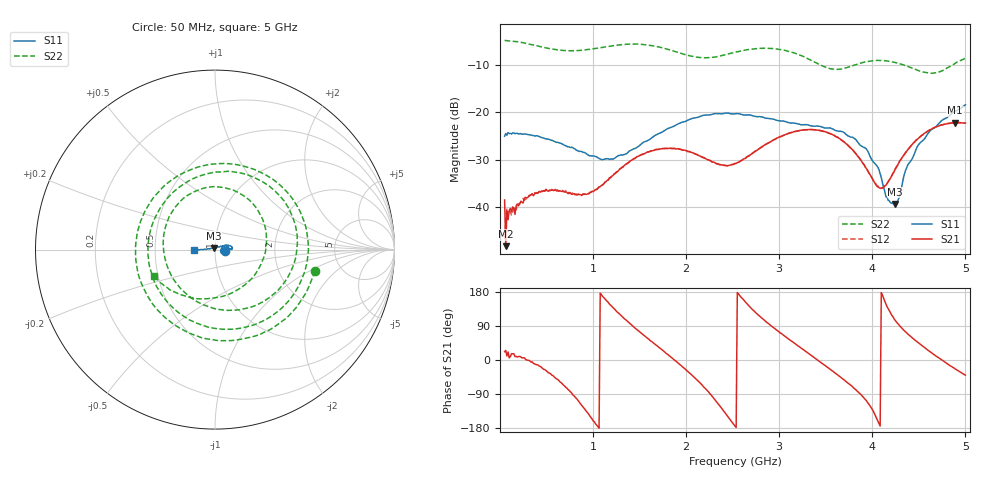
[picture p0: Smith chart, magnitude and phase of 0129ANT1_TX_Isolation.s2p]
! MASWSS0129 de-embedded Sparameters using port extention method. ANT1 to TX Isolation using 3 volt control
! 100pF blocking capacitor
! Sample board 1000013136
# Hz  S  DB  R  50
! Freq  S11  S21  S12  S22
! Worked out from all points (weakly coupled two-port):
!   401 points, 50 MHz to 5 GHz, reference 50 ohm
!   highest |S21| = -22.22 dB at 4.889 GHz (marker M1); lowest = -48.2 dB at 62.38 MHz (marker M2)
!   lowest |S11| = -39.3 dB at 4.245 GHz (marker M3), VSWR 1.02, Z = 49.3 + j0.817 ohm
!   |S11| at or under -10 dB: start of sweep to end of sweep
!   |S22| runs from -11.8 to -4.9 dB; largest |S21 - S12| = 0.009
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5e7  -25.07 -6.4  -38.48 21.8  -46.68 -19.8  -4.91 -12.0
6.2375e7  -24.50 -3.5  -48.21 25.2  -42.16 8.2  -4.94 -14.8
2.48e8  -24.63 -12.8  -39.14 5.6  -38.17 5.5  -5.41 -58.7
4.08875e8  -25.06 -18.4  -37.04 -13.3  -36.95 -14.3  -6.06 -98.4
6.44e8  -26.52 -26.4  -36.55 -57.7  -36.51 -57.0  -6.94 -159.2
8.79125e8  -28.31 -27.3  -37.42 -119.8  -37.55 -119.2  -6.96 140.1
1.12663e9  -29.90 -12.4  -34.75 161.5  -34.86 162.2  -6.29 80.7
1.3865e9  -28.25 12.1  -30.50 98.5  -30.52 98.1  -5.69 22.1
1.70825e9  -24.50 23.0  -27.80 33.4  -27.77 32.8  -6.30 -51.3
1.90625e9  -22.57 19.0  -27.69 -6.5  -27.70 -6.8  -7.41 -100.4
2.14138e9  -20.98 12.2  -29.17 -58.5  -29.12 -59.0  -8.48 -165.2
2.525e9  -20.34 2.7  -30.81 -174.0  -30.83 -173.7  -7.40 94.4
2.723e9  -20.81 1.3  -28.53 130.8  -28.47 130.7  -6.71 54.3
2.95813e9  -21.63 3.0  -25.67 81.7  -25.67 81.5  -6.66 9.4
3.35413e9  -22.95 13.9  -23.66 10.3  -23.69 10.3  -9.20 -77.6
3.72538e9  -24.80 23.5  -26.74 -58.3  -26.72 -58.3  -10.63 167.6
4.0595e9  -31.59 34.0  -35.74 -160.4  -35.57 -160.3  -9.09 91.2
4.18325e9  -38.68 65.2  -34.28 129.6  -34.28 129.6  -9.33 65.9
4.24513e9  -39.30 130.2  -32.04 105.0  -31.98 104.9  -9.55 52.6
4.49263e9  -26.98 175.5  -25.56 45.8  -25.53 45.6  -11.23 -10.0
4.88863e9  -19.86 -178.9  -22.22 -23.3  -22.23 -23.4  -9.76 -132.9
5e9  -18.46 -179.6  -22.30 -40.2  -22.32 -40.7  -8.65 -156.2
